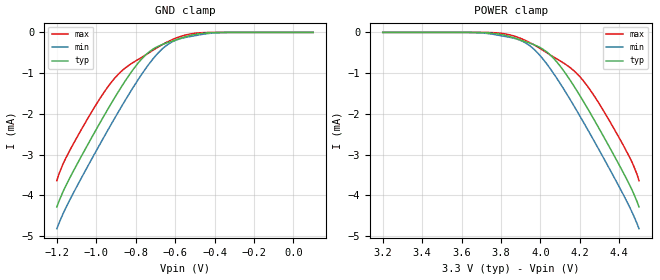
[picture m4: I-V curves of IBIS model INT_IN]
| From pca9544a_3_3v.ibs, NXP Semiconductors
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[Model]   INT_IN
Model_type Input
Vinh=2.1
Vinl=0.9
C_comp   0.5p   0.5p   0.5p
[Temperature Range] 27   85   -40
[Voltage Range]   3.3   2.97   3.63
[POWER Clamp Reference]3.3   2.97   3.63
[GND Clamp Reference]0   0   0
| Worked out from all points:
|   GND clamp passes 1 mA (typ) near -0.83 V on its own axis
[GND Clamp]
-1.2V     -4.288mA   -4.821mA   -3.642mA
-1.17V    -3.927mA   -4.471mA   -3.246mA
-1.11V    -3.352mA   -3.889mA   -2.683mA
-1V       -2.383mA   -2.909mA   -1.767mA
-920mV    -1.713mA   -2.221mA   -1.203mA
-860mV    -1.243mA   -1.724mA   -901.9uA
-770mV    -654.5uA   -1.033mA   -614.4uA
-710mV    -405uA     -638uA     -431uA
-650mV    -271.1uA   -343.2uA   -260.8uA
-540mV    -96.45uA   -116.4uA   -55.76uA
-410mV    -6.277uA   -17.26uA   -938nA
100mV     774fA      7.819pA    302.5fA
[POWER Clamp]
3.2V      774fA      7.819pA    302.5fA
3.71V     -6.277uA   -17.26uA   -938nA
3.84V     -96.45uA   -116.4uA   -55.76uA
3.95V     -271.1uA   -343.2uA   -260.8uA
4.01V     -405uA     -638uA     -431uA
4.07V     -654.5uA   -1.033mA   -614.4uA
4.16V     -1.243mA   -1.724mA   -901.9uA
4.22V     -1.713mA   -2.221mA   -1.203mA
4.3V      -2.383mA   -2.909mA   -1.767mA
4.41V     -3.352mA   -3.889mA   -2.683mA
4.47V     -3.927mA   -4.471mA   -3.246mA
4.5V      -4.288mA   -4.821mA   -3.642mA
